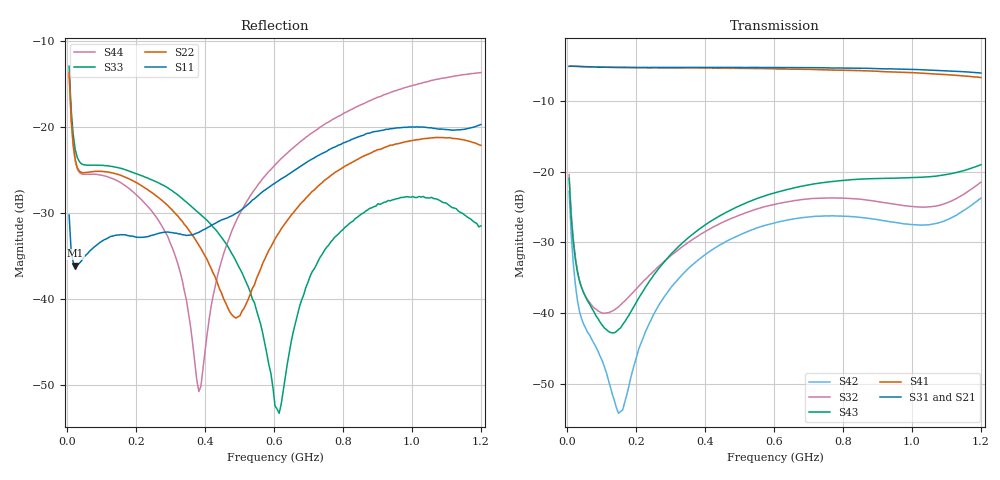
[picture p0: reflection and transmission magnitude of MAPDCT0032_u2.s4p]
#	MHz	S	dB	R	75
!FREQ	R1	I1	R2	I2	R3	I3	R4	I4
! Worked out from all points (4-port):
!   201 points, 5 MHz to 1.2 GHz, reference 75 ohm
!   strongest paths, dB at 5 MHz, 303.8 MHz, 602.5 MHz, 901.2 MHz, 1.2 GHz:
!     S31: -5.1, -5.3, -5.3, -5.4, -6.0
!     S21: -5.1, -5.3, -5.4, -5.7, -6.3
!     S41: -5.1, -5.3, -5.4, -5.8, -6.7
!     S43: -21.0, -31.5, -23.0, -21.0, -19.0
!     S32: -20.4, -31.8, -24.6, -24.2, -21.5
!     S42: -22.8, -36.2, -27.2, -26.8, -23.8
!   lowest |S11| = -36.1 dB at 22.93 MHz (marker M1), VSWR 1.03, Z = 72.7 + j0.455 ohm
!   |S11| at or under -10 dB: start of sweep to end of sweep
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5  -30.25 128.9  -5.08 0.7  -5.10 0.7  -5.10 0.7
   -5.09 0.7  -13.70 129.4  -20.48 -49.2  -22.88 -61.6
   -5.10 0.7  -20.43 -49.2  -12.96 132.9  -20.99 -50.1
   -5.10 0.7  -22.80 -61.6  -20.97 -49.9  -13.97 129.0
22.925  -36.14 168.4  -5.08 -2.5  -5.09 -2.6  -5.09 -2.6
        -5.09 -2.5  -23.85 140.1  -31.97 -58.5  -35.95 -71.5
        -5.10 -2.6  -32.01 -58.7  -22.67 139.3  -32.39 -57.7
        -5.09 -2.6  -35.89 -71.5  -32.38 -57.9  -24.04 140.3
148.4  -32.57 165.8  -5.25 -15.8  -5.24 -16.6  -5.25 -16.4
       -5.25 -15.8  -25.55 164.2  -39.10 34.1  -54.00 23.6
       -5.25 -16.7  -39.15 34.2  -24.76 157.7  -42.38 39.0
       -5.26 -16.4  -54.22 25.4  -42.35 39.1  -26.35 159.2
381.425  -32.26 92.6  -5.31 -40.1  -5.24 -42.3  -5.33 -41.6
         -5.32 -40.2  -33.76 154.3  -29.01 66.8  -32.42 92.7
         -5.25 -42.4  -29.04 66.8  -30.00 131.6  -28.19 80.6
         -5.33 -41.6  -32.44 92.8  -28.18 80.7  -50.75 58.4
614.45  -26.22 10.8  -5.42 -66.5  -5.27 -70.2  -5.46 -68.4
        -5.41 -66.6  -32.27 -82.5  -24.49 53.2  -27.11 68.7
        -5.27 -70.3  -24.50 53.1  -53.28 22.4  -22.84 63.0
        -5.46 -68.5  -27.10 68.7  -22.84 62.9  -23.95 -53.0
805.65  -21.81 -39.4  -5.55 -90.2  -5.34 -95.0  -5.67 -92.0
        -5.56 -90.3  -24.57 -85.3  -23.76 42.0  -26.33 54.2
        -5.34 -95.1  -23.77 41.9  -31.67 -73.3  -21.24 50.2
        -5.66 -92.1  -26.31 54.2  -21.23 50.2  -18.35 -66.0
1200  -19.73 178.2  -6.29 -151.0  -6.06 -157.6  -6.72 -149.5
      -6.27 -151.1  -22.16 -107.5  -21.50 78.4  -23.81 89.7
      -6.04 -157.7  -21.50 78.1  -31.52 -71.5  -19.07 57.8
      -6.68 -149.7  -23.75 89.3  -19.02 57.4  -13.70 -87.1
